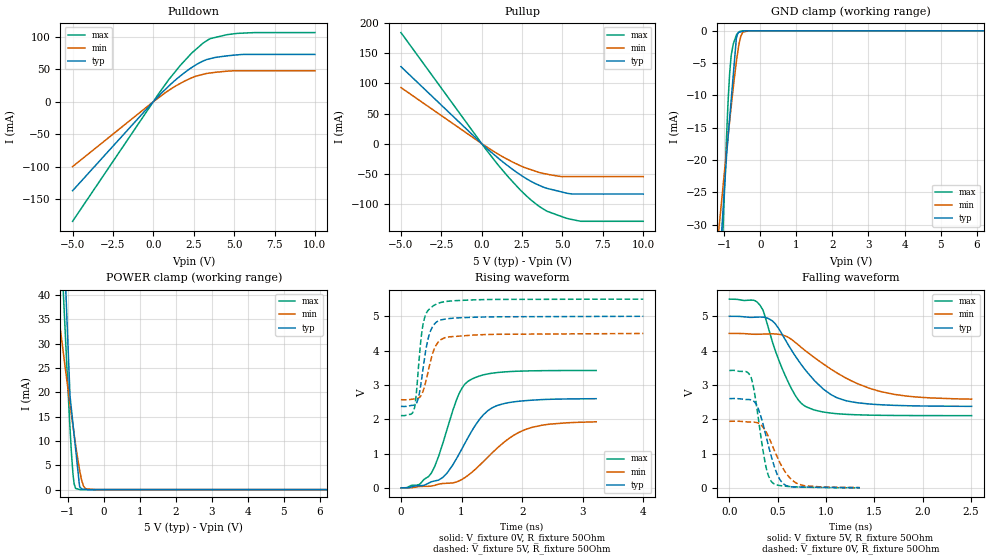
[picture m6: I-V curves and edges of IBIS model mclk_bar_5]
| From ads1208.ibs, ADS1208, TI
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|   mclk_bar_5 Model
[Model]   mclk_bar_5
Model_type   I/O
Polarity   Non-Inverting
Enable   Active-Low
Vinl = 1.5
Vinh = 3.5
Vmeas = 2.5
Vref = 2.5
Cref = 30pF
Rref = 50
|   typ   min   max
|   (nom PVT)   (fast PVT)   (slow PVT)
|C_comp from frequency sweep method (F=10MHz)
|Average
C_comp   1.694e-12   1.635e-12   1.799e-12
|ON state : BUFFER OUTPUT TURNED HIGH
|C_comp   1.912e-12   1.895e-12   1.959e-12
|OFF state: BUFFER IN HIGH IMPEDANCE
|C_comp   1.492e-12   1.357e-12   1.638e-12
|C_comp from LC tank measurement(L=1nH)
|Average
|Resonant Frequency(Hz)   5.730e+09   5.960e+09   4.975e+09
|C_comp   7.741e-13   7.179e-13   1.027e-12
|ON state : BUFFER OUTPUT TURNED HIGH
|Resonant Frequency(Hz)   5.890e+09   6.220e+09   5.130e+09
|C_comp   7.309e-13   6.554e-13   9.635e-13
|OFF state: BUFFER IN HIGH IMPEDANCE
|Resonant Frequency(Hz)   5.570e+09   5.700e+09   4.820e+09
|C_comp   8.173e-13   7.804e-13   1.091e-12
| Where nom  PVT is Nominal Process, 5V, 35C
|   Fast PVT is Strong Process,  5.5V, -40C
|   Slow PVT is Weak Process,   4.5V, 95C
[Model Spec]
|Subparameter   typ   min   max
Vinh   3.5   3.15   3.85
Vinl   1.5   1.35   1.65
[Voltage Range]   5   4.5   5.5
|Ambient Temperature   25   85   -40
|Junction Temperature
[Temperature Range]   35   95   -40
[Pullup Reference]   5   4.5   5.5
[Pulldown Reference]   0   0   0
[Power Clamp Reference]   5   4.5   5.5
[GND Clamp Reference]   0   0   0
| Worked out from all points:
|   slope of the pulldown table from 0 to 0.75 V, typ, clamps not added: 39.3 ohm
|   slope of the pullup table from 0 to 0.75 V, typ, clamps not added: 41.7 ohm
|   GND clamp passes 1 mA (typ) near -0.66 V on its own axis
|   POWER clamp passes 1 mA (typ) near -0.67 V on its own axis
|   falling waveform, V_fixture 5V, R_fixture 50Ohm: 20-80 % time 418ps typ, 655ps min, 277ps max; typ from 5 V to 2.38 V
|   rising waveform, V_fixture 0V, R_fixture 50Ohm: 20-80 % time 539ps typ, 746ps min, 387ps max; typ from 0 V to 2.6 V
|   rising waveform, V_fixture 5V, R_fixture 50Ohm: 20-80 % time 151ps typ, 178ps min, 116ps max; typ from 2.37 V to 5 V
|   falling waveform, V_fixture 0V, R_fixture 50Ohm: 20-80 % time 151ps typ, 202ps min, 112ps max; typ from 2.6 V to 0.008 V
[Pulldown]
|   Voltage   I(typ)   I(min)   I(max)
-5V       -136.9mA   -99.87mA   -183.9mA
77.86fV   19.75pA    27.7pA     17.77pA
946mV     23.71mA    17.25mA    33.62mA
1.672V    39.5mA     28.09mA    55.86mA
2.376V    52.56mA    36.74mA    74.75mA
3.08V     62.55mA    42.08mA    90.1mA
3.547V    66.31mA    44.22mA    97.15mA
4.559V    70.44mA    46.85mA    103mA
5.192V    71.96mA    47.49mA    105mA
6.309V    72.65mA    47.49mA    106.3mA
10V       72.65mA    47.49mA    106.3mA
[GND Clamp]
|   Voltage   I(typ)   I(min)   I(max)
-5V       -394.4mA   -259.4mA   -706.1mA
-1.14V    -36.54mA   -29.89mA   -46.73mA
-1.062V   -29.79mA   -25.42mA   -34.23mA
-981mV    -22.87mA   -20.83mA   -22.15mA
-891mV    -15.98mA   -15.91mA   -10.22mA
-852.5mV  -13.42mA   -13.85mA   -6.436mA
-814mV    -10.85mA   -11.87mA   -3.953mA
-753.5mV  -6.815mA   -8.788mA   -2.029mA
-670mV    -1.247mA   -4.869mA   -713.1uA
-544.5mV  -148.8uA   -820.8uA   -42.56uA
-301.5mV  -967.1nA   -791nA     -1.429uA
10V       0A         0A         0A
[Pullup]
|   Voltage   I(typ)   I(min)   I(max)
-5V       127.9mA    93.14mA    184.5mA
77.86fV   -42.66pA   -55.87pA   -36.17pA
968mV     -22.94mA   -16.73mA   -34mA
2.376V    -51.63mA   -36.65mA   -76.79mA
3.08V     -63.19mA   -43.68mA   -94.42mA
3.547V    -69.23mA   -47.93mA   -104.2mA
4.026V    -74.33mA   -50.74mA   -112.3mA
5.192V    -82.01mA   -54.85mA   -123.7mA
5.59V     -83.82mA   -54.85mA   -126.2mA
6.127V    -83.82mA   -54.85mA   -129.2mA
10V       -83.82mA   -54.85mA   -129.2mA
[POWER Clamp]
|   Voltage   I(typ)   I(min)   I(max)
-5V       1.976A     264.6mA    701.4mA
-1.373V   142.6mA    42.89mA    81.75mA
-1.305V   115mA      38.9mA     70.75mA
-1.14V    57.58mA    29.32mA    43.86mA
-1.111V   52.16mA    27.64mA    39.13mA
-1.018V   34.7mA     22.21mA    24.6mA
-935mV    19.3mA     17.54mA    12.68mA
-852.5mV  13.51mA    13.08mA    3.254mA
-781mV    8.493mA    9.332mA    247.2uA
-670mV    706.5uA    4.07mA     21.59uA
-508.5mV  34.25uA    187.8uA    111.4nA
10V       0A         0A         0A
[Ramp]
R_load = 50
|   typ   min   max
dV/dt_r   1.56052/5.36974e-10   1.16224/7.52904e-10   2.0529/3.86147e-10
dV/dt_f   1.57565/4.19306e-10   1.15831/6.62638e-10   2.03632/2.76297e-10
[Falling Waveform]
V_fixture = 5V
V_fixture_min = 4.5V
V_fixture_max = 5.5V
R_fixture = 50Ohm
|   Time   V(typ)   V(min)   V(max)
0s        5V         4.5V       5.5V
318ps     4.979V     4.478V     5.323V
464ps     4.818V     4.488V     4.099V
596ps     4.237V     4.409V     3.166V
718ps     3.699V     4.159V     2.55V
799ps     3.395V     3.972V     2.359V
1.046ns   2.731V     3.472V     2.182V
1.219ns   2.535V     3.184V     2.144V
1.703ns   2.407V     2.728V     2.112V
2.508ns   2.378V     2.587V     2.107V
[Rising Waveform]
V_fixture = 0V
V_fixture_min = 0V
V_fixture_max = 0V
R_fixture = 50Ohm
|   Time   V(typ)   V(min)   V(max)
0s        916.4pV    1.349nV    889.3pV
296ps     61.82mV    36.6mV     95.16mV
503ps     177.5mV    51.21mV    434.3mV
696ps     310.7mV    128.4mV    1.325V
940ps     923.2mV    187.7mV    2.665V
1.108ns   1.468V     364.9mV    3.106V
1.36ns    2.128V     765.9mV    3.293V
1.611ns   2.413V     1.194V     3.364V
2.159ns   2.555V     1.761V     3.41V
3.222ns   2.598V     1.925V     3.421V
[Rising Waveform]
V_fixture = 5V
V_fixture_min = 4.5V
V_fixture_max = 5.5V
R_fixture = 50Ohm
|   Time   V(typ)   V(min)   V(max)
0s        2.374V     2.568V     2.106V
213ps     2.41V      2.59V      2.262V
243ps     2.44V      2.596V     2.567V
289ps     2.629V     2.615V     3.506V
330ps     3.027V     2.684V     4.318V
370ps     3.537V     2.842V     4.808V
462ps     4.437V     3.503V     5.199V
587ps     4.834V     4.177V     5.356V
1.174ns   4.97V      4.449V     5.477V
3.999ns   5V         4.499V     5.5V
[Falling Waveform]
V_fixture = 0V
V_fixture_min = 0V
V_fixture_max = 0V
R_fixture = 50Ohm
|   Time   V(typ)   V(min)   V(max)
0s        2.602V     1.941V     3.422V
171ps     2.577V     1.928V     3.391V
225ps     2.566V     1.92V      3.218V
293ps     2.355V     1.898V     2.17V
380ps     1.517V     1.636V     606.9mV
443ps     835.6mV    1.252V     163.4mV
496ps     392.4mV    904.2mV    84.9mV
551ps     147.7mV    592.5mV    59.84mV
692ps     27.38mV    145.5mV    31.9mV
1.352ns   7.936mV    11.88mV    3.541mV
